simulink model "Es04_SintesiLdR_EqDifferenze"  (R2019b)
settings: Solver=ode4  StartTime=0.0  StopTime=15  FixedStep=0.0001  RelTol=1e-3
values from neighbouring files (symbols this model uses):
  Tc = 1    [Es04_svolgimento.m]
undefined symbols (not defined in the file or in its folder): k

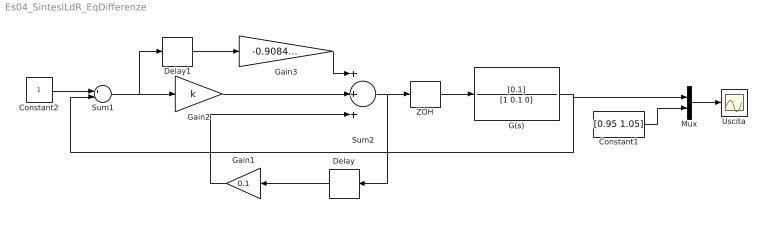
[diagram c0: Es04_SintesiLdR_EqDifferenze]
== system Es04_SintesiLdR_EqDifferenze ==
  Constant1 : Constant  Value=[0.95 1.05]
  Constant2 : Constant
  Delay : Delay  DelayLength=1  SampleTime=Tc
  Delay1 : Delay  DelayLength=1  SampleTime=Tc
  G(s) : TransferFcn  Numerator=[0.1]  Denominator=[1 0.1 0]
  Gain1 : Gain  Gain=0.1
  Gain2 : Gain  Gain=k
  Gain3 : Gain  Gain=-0.9084*k
  Mux : Mux  Inputs=2
  Sum1 : Sum  Inputs=+-
  Sum2 : Sum  Inputs=+++
  Uscita : Scope
  ZOH : ZeroOrderHold  SampleTime=Tc
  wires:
  Mux/1 -> Uscita/1
  Sum2/1 -> Delay/1, ZOH/1
  Constant2/1 -> Sum1/1
  G(s)/1 -> Sum1/2, Mux/1
  Sum1/1 -> Gain2/1, Delay1/1
  ZOH/1 -> G(s)/1
  Delay/1 -> Gain1/1
  Gain1/1 -> Sum2/3
  Gain2/1 -> Sum2/2
  Gain3/1 -> Sum2/1
  Delay1/1 -> Gain3/1
  Constant1/1 -> Mux/2
